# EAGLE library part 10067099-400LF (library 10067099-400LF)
Check availability
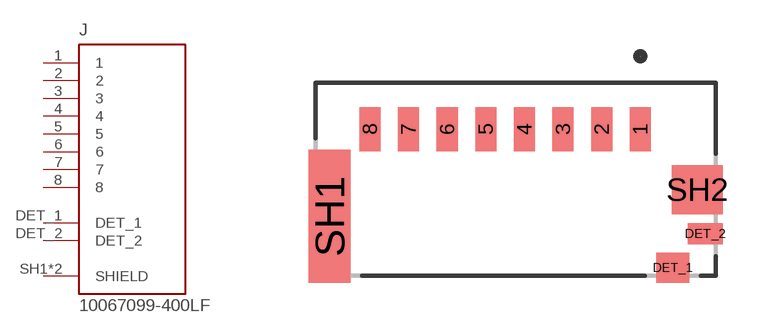
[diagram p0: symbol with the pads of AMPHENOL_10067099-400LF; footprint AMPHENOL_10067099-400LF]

Designator prefix J

## 10067099-400LF (Availability: In Stock; Check_prices: https://www.snapeda.com/parts/10067099-400LF/Amphenol+FCI/view-part/?ref=eda; Description: 3.05mm Height with protection T-Flash Connector; MF: Amphenol ICC (FCI); MP: 10067099-400LF; Package: None; Price: None; Purchase-URL: https://www.snapeda.com/api/url_track_click_mouser/?unipart_id=5672934&manufacturer=Amphenol ICC (FCI)&part_name=10067099-400LF&search_term=None; SnapEDA_Link: https://www.snapeda.com/parts/10067099-400LF/Amphenol+FCI/view-part/?ref=snap)  [AMPHENOL_10067099-400LF]
1  1  pas
2  2  pas
3  3  pas
4  4  pas
5  5  pas
6  6  pas
7  7  pas
8  8  pas
DET_1  DET_1  pas
DET_2  DET_2  pas
SH1  SHIELD  pas
SH2  SHIELD  pas

## Footprint AMPHENOL_10067099-400LF (pad centres in mm)
smd 0.6 x 1.25: 1 3.55,1.425; 2 2.45,1.425; 3 1.35,1.425; 4 0.25,1.425; 5 -0.85,1.425; 6 -1.95,1.425; 7 -3.05,1.425; 8 -4.15,1.425
smd 0.95 x 0.85: DET_1 4.475,-2.525
smd 1 x 0.6: DET_2 5.4,-1.55
smd 1.2 x 3.79: SH1 -5.3,-1.055
smd 1.45 x 1.4: SH2 5.175,-0.3

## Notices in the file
This work is licensed under a Creative Commons Attribution-ShareAlike 4.0 International License (CC BY-SA) with Design Exception 1.0
